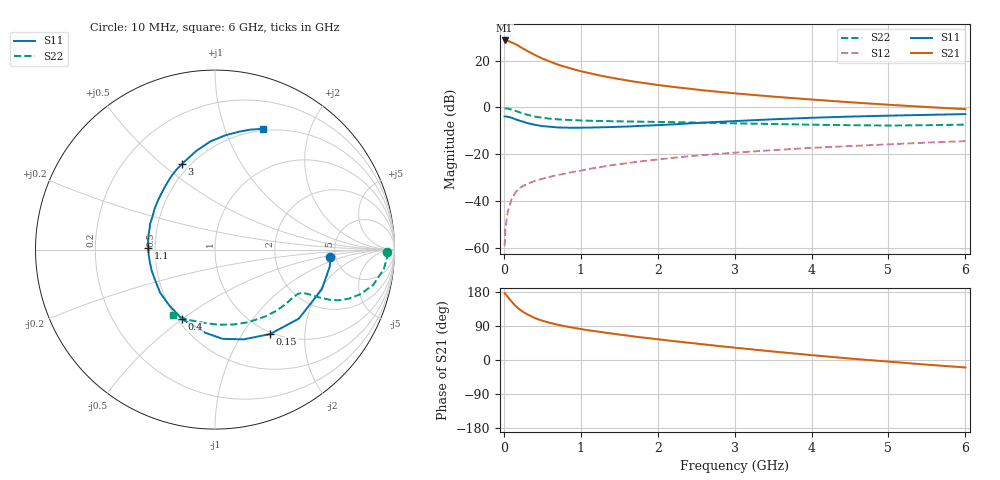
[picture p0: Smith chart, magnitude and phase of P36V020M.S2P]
! SIEMENS Small Signal Semiconductors
! BFP181
! Si NPN RF Bipolar Junction Transistor in SOT143
! VCE = 6 V  IC = 20 mA
! Common Emitter S-Parameters:  March  1996
# GHz  S  MA  R  50
!  f  S11  S21  S12  S22
! GHz  MAG  ANG  MAG  ANG  MAG  ANG  MAG  ANG
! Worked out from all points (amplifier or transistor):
!   36 points, 10 MHz to 6 GHz, reference 50 ohm
!   highest |S21| = 28.6 dB at 10 MHz (marker M1)
!   |S21| within 3 dB of that: start of sweep to 226.2 MHz
!   unconditionally stable (mu >= 1): 762.5 MHz to end of sweep
!   at 250 MHz: K = 0.49, MSG = 29.3 dB, |S12| = -33.5 dB
!   at 1.4 GHz: K = 1.18, MAG = 16.1 dB, |S12| = -24.7 dB
!   at 6 GHz: K = 1.01, MAG = 6.1 dB, |S12| = -14.3 dB
!   S11 on the Smith chart (normalised r, x): 10 MHz: 4.50, -0.67; 150 MHz: 0.98, -1.34; 400 MHz: 0.53, -0.50; 1.1 GHz: 0.46, +0.01; 3 GHz: 0.45, +0.59; 6 GHz: 0.48, +1.36
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0.01  0.6429 -3.9  26.93 176.6  0.0011 72.1  0.9584 -0.9
0.02  0.6466 -8.3  26.93 174.5  0.0025 77.9  0.9612 -2.4
0.05  0.6348 -20.3  26.46 166.5  0.0059 81.3  0.9464 -6.6
0.1  0.6054 -39.4  24.53 154.2  0.011 72.1  0.9039 -12.5
0.15  0.5617 -56.9  22.47 143.2  0.0153 65.8  0.8482 -17.0
0.2  0.5252 -72.2  20.25 134.3  0.0189 62.5  0.7933 -20.2
0.25  0.4993 -85.0  18.06 126.8  0.0212 58.2  0.744 -22.3
0.3  0.4672 -96.4  16.25 121.0  0.0232 56.9  0.7031 -23.5
0.4  0.4284 -115.4  13.28 110.9  0.0271 55.3  0.643 -24.6
0.5  0.401 -130.0  11.07 103.7  0.0301 53.5  0.6029 -25.1
0.6  0.3886 -142.0  9.547 98.0  0.0332 54.2  0.5767 -25.5
0.7  0.3752 -152.1  8.25 93.2  0.0363 54.4  0.559 -25.9
0.9  0.3698 -168.5  6.6 85.3  0.0421 54.9  0.5366 -26.9
1.1  0.3723 178.6  5.47 78.4  0.0486 55.6  0.5224 -28.4
1.3  0.3792 167.6  4.625 72.7  0.0552 55.2  0.5138 -30.5
1.6  0.3923 153.7  3.786 64.6  0.065 54.5  0.5036 -33.9
2.2  0.4362 132.3  2.75 50.0  0.0844 51.7  0.4865 -42.5
3  0.5125 110.9  2.007 32.6  0.1086 46.0  0.4591 -56.0
3.5  0.5604 100.6  1.706 22.4  0.1231 42.2  0.4447 -65.7
4.5  0.6398 84.8  1.294 3.8  0.1503 34.0  0.4188 -87.8
5.5  0.6962 73.7  1.024 -12.3  0.1783 26.6  0.4188 -111.1
6  0.7235 68.5  0.923 -19.7  0.1917 22.2  0.4312 -122.8
